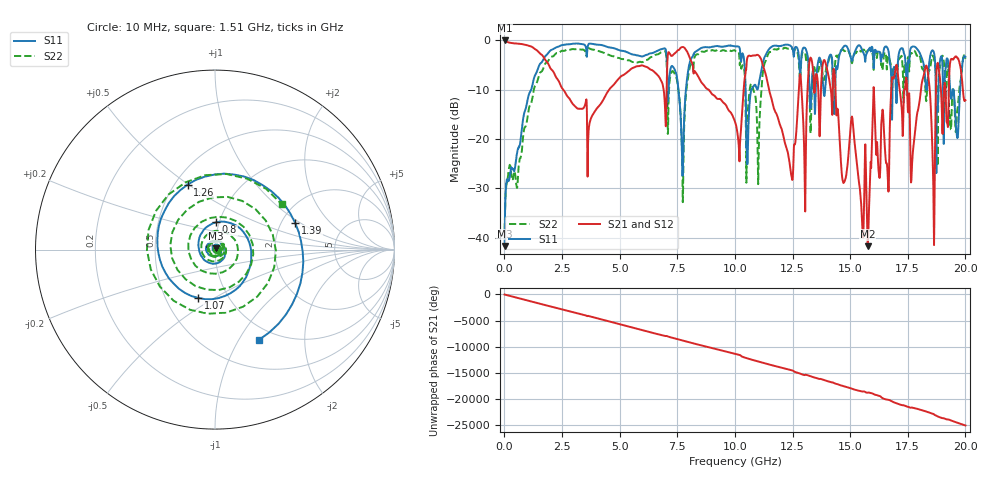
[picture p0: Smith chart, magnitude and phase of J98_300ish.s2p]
!Keysight Technologies,N5222A,MY51421036,A.10.65.16
!Date: Friday, March 31, 2023 15:21:05
!Correction: S11(Full 2 Port(1,2))
!S21(Full 2 Port(1,2))
!S12(Full 2 Port(1,2))
!S22(Full 2 Port(1,2))
!S2P File: Measurements: S11, S21, S12, S22:
# Hz S  dB  R 50
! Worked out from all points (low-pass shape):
!   2000 points, 10 MHz to 20 GHz, reference 50 ohm
!   highest |S21| = -0.02 dB at 10 MHz (marker M1); lowest = -41.7 dB at 15.76 GHz (marker M2)
!   |S21| within 3 dB of the highest: start of sweep to 1.645 GHz; 7.305 GHz to 7.998 GHz (692.5 MHz wide, 9.05 % of centre)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
!   lowest |S11| = -41.7 dB at 10 MHz (marker M3), VSWR 1.02, Z = 50.5 + j0.673 ohm
!   |S11| at or under -10 dB: start of sweep to 1.161 GHz; 7.549 GHz to 7.874 GHz (325.3 MHz wide, 4.22 % of centre); 19.48 GHz to 19.77 GHz (288.9 MHz wide, 1.47 % of centre)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
!   |S22| runs from -38.5 to -1.5 dB; largest |S21 - S12| = 0.013
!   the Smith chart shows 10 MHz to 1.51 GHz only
!   S11 on the Smith chart (normalised r, x): 10 MHz: 1.01, +0.01; 800 MHz: 0.97, +0.30; 1.07 GHz: 0.73, -0.42; 1.26 GHz: 0.58, +0.50; 1.39 GHz: 2.36, +0.91; 1.51 GHz: 0.84, -1.22
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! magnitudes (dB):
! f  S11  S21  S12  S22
! 10 MHz  -41.7  0.0  -0.1  -38.5
! 800 MHz  -16.4  -0.8  -0.8  -20.1
! 1.07 GHz  -10.9  -1.1  -1.1  -13.6
! 1.26 GHz  -8.1  -1.5  -1.5  -10.4
! 1.39 GHz  -6.5  -1.9  -1.9  -8.7
! 1.51 GHz  -5.0  -2.5  -2.5  -6.9
! 3.35 GHz  -0.7  -13.9  -13.8  -1.9
! 6.68 GHz  -2.0  -7.2  -7.2  -2.8
! 7.73 GHz  -27.5  -1.3  -1.3  -29.5
! 10.01 GHz  -1.2  -16.6  -16.6  -2.1
! 11.03 GHz  -9.1  -3.1  -3.1  -23.1
! 12.44 GHz  -1.2  -27.2  -27.1  -1.6
! 13.34 GHz  -8.3  -4.2  -4.2  -10.0
! 15.76 GHz  -2.2  -41.7  -41.1  -2.0
! 16.02 GHz  -5.7  -9.5  -9.5  -6.0
! 16.67 GHz  -2.3  -30.5  -30.6  -3.2
! 16.97 GHz  -7.6  -5.8  -5.7  -8.3
! 17.7 GHz  -1.3  -24.0  -23.9  -2.4
! 18.27 GHz  -8.5  -5.3  -5.3  -10.6
! 18.6 GHz  -2.1  -27.8  -27.8  -3.2
! 18.82 GHz  -11.6  -4.9  -4.9  -12.3
! 20 GHz  -3.3  -12.1  -12.1  -3.7
